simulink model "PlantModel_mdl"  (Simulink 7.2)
settings: Solver=ode45  StartTime=0.0  StopTime=10  RelTol=1e-3
InitFcn:
  | s = tf('s');
  | G_plant = (101*s + 808)/(s^3 + 6*s^2 + 109*s + 404);
  | Gd_plant = tf(c2d(G_plant,Ts,'zoh'))
  | [B_plant,A_plant] = tfdata(Gd_plant,'v');
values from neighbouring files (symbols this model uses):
  Ts = 0.01    [Esercitazione03.m]
undefined symbols (not defined in the file or in its folder): A_plant, polyval
libraries: simulink x1, cstblocks x1

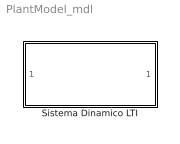
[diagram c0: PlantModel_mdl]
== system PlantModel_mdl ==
  Sistema Dinamico LTI : Subsystem

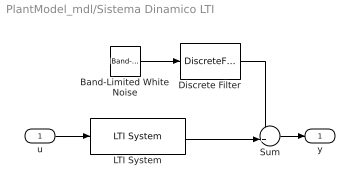
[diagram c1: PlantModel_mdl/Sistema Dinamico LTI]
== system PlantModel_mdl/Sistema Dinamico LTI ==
  u : Inport
  Band-Limited White Noise : simulink/Sources/Band-Limited White Noise  SystemSampleTime=-1  Cov=0.0001  Ts=Ts  seed=[23341]
  Discrete Filter : DiscreteFilter  Numerator=polyval(A_plant,1)*[1]  Denominator=A_plant  SampleTime=Ts
  LTI System : cstblocks/LTI System  SystemSampleTime=-1  sys=Gd_plant  IC=[]
  Sum : Sum  Inputs=++|  OutDataType=sfix(16)  OutScaling=2^0
  y : Outport
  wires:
  LTI System/1 -> Sum/2
  u/1 -> LTI System/1
  Sum/1 -> y/1
  Band-Limited White Noise/1 -> Discrete Filter/1
  Discrete Filter/1 -> Sum/1
